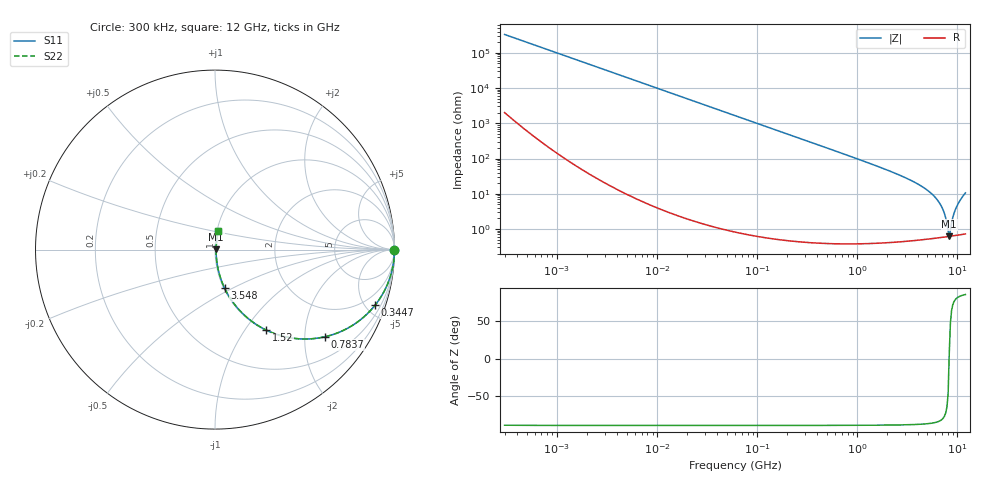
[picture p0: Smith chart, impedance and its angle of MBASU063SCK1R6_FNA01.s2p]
! MBASU063SCK1R6_FNA01  S-PARAMETER MODEL  ( Standard Model )
! Model Generated by TAIYO YUDEN Corporation (http://www.ty-top.com)
! Version 1.0
! TAIYO YUDEN Control No. 230609
! Copyright(c) 2023 TAIYO YUDEN CO.,LTD. All Rights Reserved.
! Product Description (link to TY-COMPAS)
! https://ds.yuden.co.jp/TYCOMPAS/or/detail?pn=MBASU063SCK1R6BFNA01&u=M
! Products Name : Multilayer Ceramic Capacitors
! Characteristics :
!  Capacitance : 1.6 [pF] , Rated Voltage : 50 [V] , TCC : CK / C0K
!  Case Size : 0.6 x 0.3 / 0.024 x 0.012 [mm/inch] , Thickness : 0.3 / 0.012 [mm/inch]
!  (Conditions: Temperature = 25 [degC] , DC Bias Voltage = 0 [V])
! External Node Assignments :
!  1  o---| |---o  2
! GND o---------o GND
! Frequency Range : 0.3MHz  -  12000MHz  [ 401 STEP ]
# MHZ S RI R 50
! Freq[MHz].  S11 Real  S11 Imag  S21 Real  S21 Imag  S12 Real  S12 Imag  S22 Real  S22 Imag
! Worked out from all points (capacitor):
!   401 points, 300 kHz to 12 GHz, reference 50 ohm
!   read as one part in series: C = 1.6 pF near 316.3 kHz
!   lowest |Z| = 622 mohm at 8.282 GHz (marker M1)
!   series resonance near 8.259 GHz, so ESL is about 230 pH
!   S11 on the Smith chart (normalised r, x): 300 kHz: open; 344.7 MHz: 1.01, -5.75; 783.7 MHz: 1.01, -2.51; 1.52 GHz: 1.01, -1.26; 3.548 GHz: 1.01, -0.46; 12 GHz: 1.01, +0.21
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0.3  1 -0.000302  1.93e-06 0.000302  1.93e-06 0.000302  1 -0.000302
1.769972  1 -0.00178  4.73e-06 0.00178  4.73e-06 0.00178  1 -0.00178
10.44266  0.9999 -0.0105  0.000115 0.0105  0.000115 0.0105  0.9999 -0.0105
60  0.9963 -0.0603  0.00367 0.0603  0.00367 0.0603  0.9963 -0.0603
151.6462  0.977 -0.1494  0.023 0.1494  0.023 0.1494  0.977 -0.1494
344.7396  0.8916 -0.3102  0.1084 0.3102  0.1084 0.3102  0.8916 -0.3102
353.9943  0.8864 -0.3167  0.1136 0.3167  0.1136 0.3167  0.8864 -0.3167
783.7017  0.6112 -0.486  0.3888 0.486  0.3888 0.486  0.6112 -0.486
1519.776  0.2859 -0.4487  0.7141 0.4487  0.7141 0.4487  0.2859 -0.4487
2088.533  0.1675 -0.3688  0.8325 0.3688  0.8325 0.3688  0.1675 -0.3688
3547.679  0.0535 -0.2152  0.9465 0.2152  0.9465 0.2152  0.0535 -0.2152
4875.354  0.0222 -0.1295  0.9778 0.1295  0.9778 0.1295  0.0222 -0.1295
6188.031  0.0104 -0.0698  0.9896 0.0698  0.9896 0.0698  0.0104 -0.0698
7064.448  0.00722 -0.0379  0.9928 0.0379  0.9928 0.0379  0.00722 -0.0379
7448.838  0.00653 -0.0253  0.9935 0.0253  0.9935 0.0253  0.00653 -0.0253
7854.144  0.00617 -0.0127  0.9938 0.0127  0.9938 0.0127  0.00617 -0.0127
8281.503  0.00614 0.000754  0.9939 -0.000754  0.9939 -0.000754  0.00614 0.000754
8503.825  0.00625 0.00685  0.9938 -0.00685  0.9938 -0.00685  0.00625 0.00685
9207.246  0.00708 0.0259  0.9929 -0.0259  0.9929 -0.0259  0.00708 0.0259
9968.853  0.00875 0.0459  0.9913 -0.0459  0.9913 -0.0459  0.00875 0.0459
11083.22  0.0128 0.0763  0.9872 -0.0763  0.9872 -0.0763  0.0128 0.0763
12000  0.0179 0.1028  0.9821 -0.1028  0.9821 -0.1028  0.0179 0.1028
